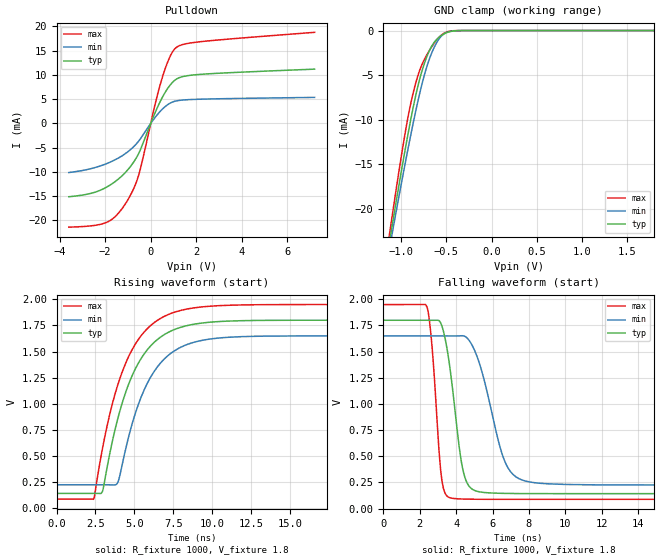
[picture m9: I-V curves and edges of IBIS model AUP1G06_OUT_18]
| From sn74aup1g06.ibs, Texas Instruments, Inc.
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[Model]   AUP1G06_OUT_18
Model_type  Open_drain
Enable   Active-Low
Vref =   1.8
Rref =   1E6
Cref =   30p
Vmeas =   0.9
| variable   typ   min   max
C_comp   1.66pF   1.41pF   1.95pF
| C_pulldown   2.06pF   1.69pF   2.56pF
| C_tri-state   1.66pF   1.41pF   1.95pF
[Temperature Range]   40   100   -40
| Ambient temperature   25   85   -40
[Voltage range]   1.8   1.65   1.95
[Pullup Reference]   1.8   1.8   1.8
[POWER Clamp Reference]   1.8   1.8   1.8
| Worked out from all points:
|   slope of the pulldown table from 0 to 0.27 V, typ, clamps not added: 88.7 ohm
|   GND clamp passes 1 mA (typ) near -0.61 V on its own axis
|   rising waveform, R_fixture 1000, V_fixture 1.8: 20-80 % time 2.24ns typ, 2.19ns min, 2.28ns max; typ from 0.142 V to 1.8 V
|   falling waveform, R_fixture 1000, V_fixture 1.8: 20-80 % time 708ps typ, 1.23ns min, 441ps max; typ from 1.8 V to 0.142 V
[GND Clamp]
| AUP1G06_OUT_18
|   Voltage   I(typ)   I(min)   I(max)
-3.6V     -193.5mA   -179.7mA   -210.2mA
-1.145V   -24.44mA   -25.11mA   -23.69mA
-1.12V    -22.9mA    -23.71mA   -21.96mA
-1.095V   -21.37mA   -22.31mA   -20.26mA
-945mV    -12.59mA   -14.19mA   -10.7mA
-840mV    -7.223mA   -8.972mA   -5.843mA
-770mV    -4.468mA   -5.927mA   -3.764mA
-695mV    -2.372mA   -3.345mA   -2.326mA
-615mV    -1.069mA   -1.462mA   -1.136mA
-540mV    -445.1uA   -477.1uA   -389.8uA
-315mV    -2.831uA   -4.161uA   -587.6nA
1.8V      150.2pA    616.6pA    31.88pA
[Pulldown]
| AUP1G06_OUT_18
|   Voltage   I(typ)   I(min)   I(max)
-3.6V     -15.12mA   -10.13mA   -21.39mA
-1.915V   -13.07mA   -8.246mA   -20.35mA
-1.485V   -11.71mA   -7.301mA   -18.84mA
-1.03V    -9.681mA   -5.933mA   -15.95mA
-725mV    -7.787mA   -4.683mA   -13.18mA
-520mV    -6.099mA   -3.59mA    -10.49mA
205mV     2.352mA    1.308mA    4.202mA
545mV     5.664mA    3.086mA    10.01mA
855mV     7.912mA    4.18mA     13.84mA
1.115V    9.087mA    4.628mA    15.61mA
2.18V     10.1mA     4.986mA    16.83mA
7.2V      11.18mA    5.355mA    18.77mA
[Ramp]
| AUP1G06_OUT_18
| variable   typ   min   max
dV/dt_r   1.00/2.24E-09   0.86/2.19E-09   1.12/2.28E-09
dV/dt_f   1.00/7.10E-10   0.86/1.23E-09   1.12/4.46E-10
R_load = 1000
[Rising Waveform]
| AUP1G06_OUT_18
R_fixture =   1000
C_fixture =   0
L_fixture =   0
V_fixture =   1.8
V_fixture_min = 1.65
V_fixture_max = 1.95
|   Time   V(typ)   V(min)   V(max)
0s        142.2mV    224.7mV    87.89mV
2.4ns     142.2mV    224.7mV    91.97mV
2.955ns   162.1mV    224.8mV    572.5mV
3.865ns   815.3mV    230.8mV    1.145V
4.65ns    1.193V     692.2mV    1.456V
5.545ns   1.458V     1.102V     1.671V
6.425ns   1.607V     1.341V     1.792V
7.48ns    1.704V     1.497V     1.871V
11.87ns   1.795V     1.642V     1.946V
35.9ns    1.8V       1.65V      1.95V
[Falling Waveform]
| AUP1G06_OUT_18
R_fixture =   1000
C_fixture =   0
L_fixture =   0
V_fixture =   1.8
V_fixture_min = 1.65
V_fixture_max = 1.95
|   Time   V(typ)   V(min)   V(max)
0s        1.8V       1.65V      1.95V
2.4ns     1.8V       1.65V      1.924V
2.675ns   1.8V       1.65V      1.545V
3.185ns   1.76V      1.65V      310.2mV
3.685ns   1.308V     1.65V      101.8mV
4.255ns   480.4mV    1.652V     91.52mV
4.66ns    225.8mV    1.619V     89.58mV
6.655ns   144.8mV    458.8mV    87.96mV
7.825ns   142.9mV    261.9mV    87.9mV
35.9ns    142.2mV    224.7mV    87.89mV
